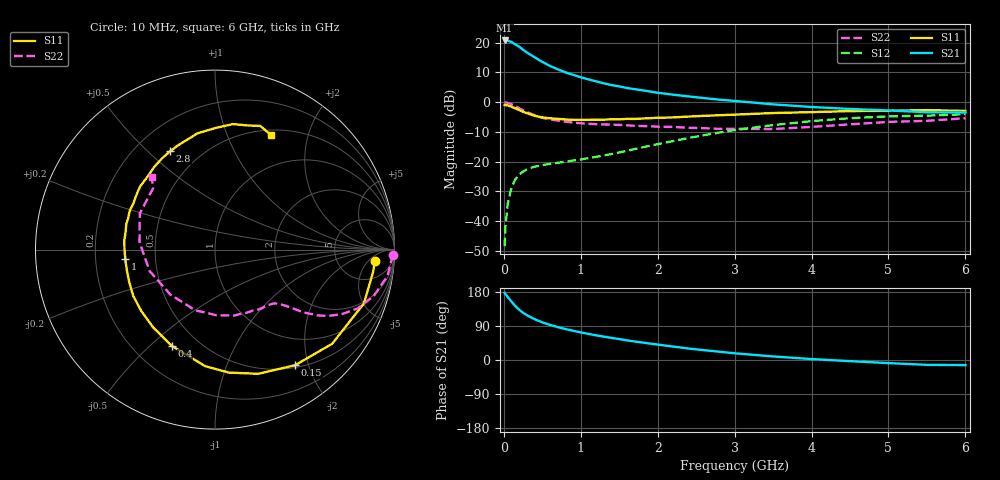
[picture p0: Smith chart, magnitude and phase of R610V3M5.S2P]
! SIEMENS Small Signal Semiconductors
! BFR193
! Si NPN RF Bipolar Junction Transistor in SOT23
! VCE = 10 V  IC = 3.5 mA
! Common Emitter S-Parameters:  May  1996
# GHz  S  MA  R  50
!  f  S11  S21  S12  S22
! GHz  MAG  ANG  MAG  ANG  MAG  ANG  MAG  ANG
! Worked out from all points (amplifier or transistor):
!   36 points, 10 MHz to 6 GHz, reference 50 ohm
!   highest |S21| = 20.7 dB at 10 MHz (marker M1)
!   |S21| within 3 dB of that: start of sweep to 243.9 MHz
!   unconditionally stable (mu >= 1): 1.021 GHz to 2.069 GHz
!   at 250 MHz: K = 0.33, MSG = 20.5 dB, |S12| = -23.3 dB
!   at 1.4 GHz: K = 1.08, MAG = 9.9 dB, |S12| = -17.4 dB
!   at 6 GHz: K = 0.97, MSG = 0.3 dB, |S12| = -4.1 dB
!   S11 on the Smith chart (normalised r, x): 10 MHz: 13, -8; 150 MHz: 0.53, -1.78; 400 MHz: 0.36, -0.59; 1 GHz: 0.33, -0.05; 2.8 GHz: 0.34, +0.59; 6 GHz: 0.56, +1.45
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0.01  0.8929 -4.0  10.86 177.4  0.0038 85.7  0.9927 -1.6
0.02  0.8897 -8.1  10.68 174.3  0.0079 84.7  0.9847 -3.4
0.05  0.8822 -19.9  10.79 166.4  0.0195 78.9  0.9723 -8.7
0.1  0.8375 -38.8  10.22 153.9  0.0368 69.6  0.9208 -16.4
0.15  0.7836 -55.3  9.298 142.0  0.0505 61.6  0.859 -22.5
0.2  0.7327 -70.8  8.526 132.6  0.0607 55.8  0.7896 -27.2
0.25  0.6894 -83.6  7.577 124.6  0.0681 51.0  0.7283 -30.5
0.3  0.6519 -94.8  6.805 118.1  0.0744 48.0  0.6807 -32.6
0.4  0.5879 -114.2  5.67 107.8  0.0822 44.1  0.6005 -35.5
0.5  0.5537 -128.5  4.733 99.3  0.0872 42.6  0.5449 -37.0
0.6  0.5345 -140.3  4.058 92.7  0.0918 42.2  0.5126 -38.1
0.8  0.5114 -159.2  3.167 81.8  0.0997 44.0  0.4702 -40.2
1  0.5029 -174.0  2.619 72.8  0.1087 47.9  0.4415 -43.0
1.1  0.5043 179.8  2.409 68.9  0.1146 50.0  0.4333 -44.9
1.3  0.5076 169.0  2.067 61.7  0.1272 53.2  0.4214 -48.6
1.6  0.5226 155.1  1.727 51.8  0.152 57.4  0.4082 -55.7
2.2  0.553 133.1  1.334 35.5  0.2216 59.5  0.3831 -73.7
2.8  0.6022 114.6  1.1 21.9  0.3081 54.9  0.3549 -98.1
3.5  0.6552 98.5  0.917 9.4  0.4112 44.5  0.3531 -134.9
4.5  0.7064 81.9  0.767 -3.0  0.5367 26.6  0.4229 174.2
5.5  0.7339 69.9  0.675 -12.8  0.5917 8.3  0.4852 135.4
6  0.711 64.1  0.67 -13.4  0.6267 3.3  0.5365 131.1
